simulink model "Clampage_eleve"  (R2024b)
settings: Solver=VariableStepAuto  StartTime=0.0  StopTime=1.5  MaxStep=1e-2  RelTol=1e-3  EnableMultiTasking=on
libraries: fl_lib x12, nesl_utility x5, simulink x2, ee_lib x2, simulink_extras x1

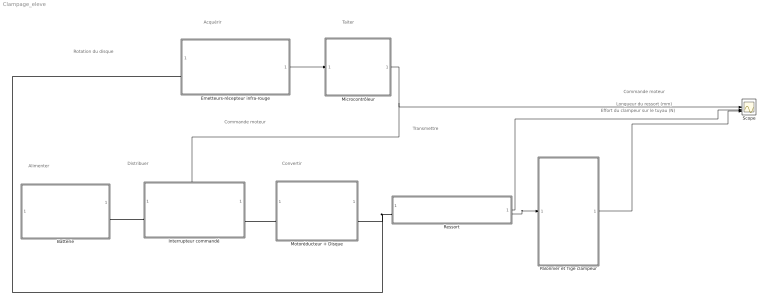
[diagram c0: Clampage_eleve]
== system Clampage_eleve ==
  note: Acquérir
  note: Longueur du ressort (mm)
  note: Effort du clampeur sur le tuyau (N)
  note: Commande moteur
  note: Taiter
  note: Convertir
  note: Alimenter
  note: Transmettre
  note: Rotation du disque
  note: Commande moteur
  note: Distribuer
  Batterie : Subsystem
  Emetteurs-récepteur infra-rouge : Subsystem
  Interrupteur commandé : Subsystem
  Microcontrôleur : Subsystem
  Motoréducteur + Disque : Subsystem  mask{V=0, R=0}
      mask prompts: V "Vitesse de rotation à vide (tr/min)"; R "Rapport de réduction"
  Palonnier et Tige clampeur : Subsystem
  Ressort : Subsystem  mask{k=0, L0=0}
      mask prompts: k "k : Raideur du ressort (N/mm)"; L0 "L0 : Longueur libre initiale du ressort (mm)"
  Scope : Scope  NumInputPorts=3
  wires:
  Ressort/2(Out3) -> Palonnier et Tige clampeur/1(In1)
  Emetteurs-récepteur infra-rouge/1(Out1) -> Microcontrôleur/1(S)
  Microcontrôleur/1(Q) -> Interrupteur commandé/1(In1), Scope/1
  Palonnier et Tige clampeur/1(Out1) -> Scope/3
  Ressort/1(Out1) -> Scope/2
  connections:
  Ressort/LConn1 -- Emetteurs-récepteur infra-rouge/LConn1 -- Motoréducteur + Disque/RConn1
  Interrupteur commandé/RConn1 -- Motoréducteur + Disque/LConn1
  Batterie/RConn1 -- Interrupteur commandé/LConn1

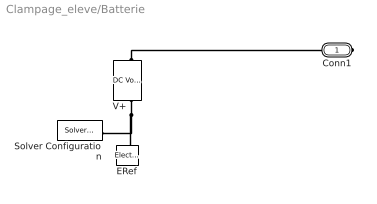
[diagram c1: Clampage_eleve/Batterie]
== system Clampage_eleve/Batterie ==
  ERef : fl_lib/Electrical/Electrical Elements/Electrical Reference
  Solver Configuration : nesl_utility/Solver Configuration  PhysicalDomain=network_engine_domain  SubClassName=solver  LeftPortType=input  RightPortType=generic  Tones=[]  Harmonics=[]  SimulateNoise=off  Profile=off  UseLocalSampling=off  EnableSwitchedLinearOptims=on  FrequencyDomain=off  UseCCode=off  RelTol=0.001  AbsTol=1e-06  MinStep=1e-09  ToWorkspace=off  RevertToSquareIcSolve=off  NumHomotopyIterations=100  PhasorMode=off  PhasorModeNumHarmonics=1  ConsistencySolver=NEWTON_FTOL  IndexReductionMethod=DerivativeReplacement  DoDC=off  ResidualTolerance=1e-9  ConsistencyTolSource=GLOBAL  ConsistencyAbsTol=0.001  ConsistencyRelTol=0.001  ConsistencyTolFactor=0.001  UseLocalSolver=off  LocalSolverChoice=NE_BACKWARD_EULER_ADVANCER  ResolveIndetEquations=on  FunctionEvalNumThread=1  LocalSolverSampleTime=.001  DoFixedCost=off  MaxNonlinIter=3  MaxModeIter=2  ComputeImpulses=off  ImpulseIterations=2  LinearAlgebra=auto  LinearAlgebraNumThread=0  EquationFormulation=NE_TIME_EF  DelaysMemoryBudget=1024  AutomaticFiltering=on  FilteringTimeConstant=0.001  PartitionStorageMethod=AS_NEEDED  PartitionMemoryBudget=1024  PartitionMethod=FAST  MultibodyUseLocalSolver=off  MultibodyLocalSolverChoice=ODE1  MultibodyLocalSolverSampleTime=0.001
  V+ : fl_lib/Electrical/Electrical Sources/DC Voltage Source  v0=12 V
  Conn1 : PMIOPort  Side=Right
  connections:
  V+/RConn1 -- ERef/LConn1 -- Solver Configuration/RConn1
  V+/LConn1 -- Conn1/RConn1

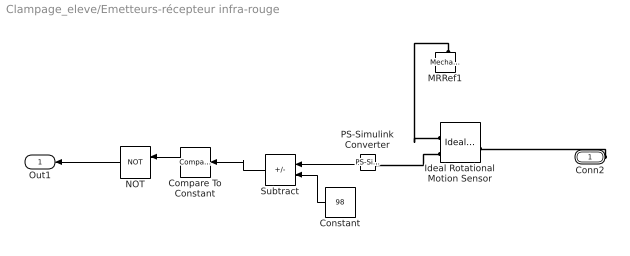
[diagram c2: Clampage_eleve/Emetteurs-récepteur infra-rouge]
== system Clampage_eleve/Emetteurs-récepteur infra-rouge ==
  Compare To Constant : simulink/Logic and Bit Operations/Compare To Constant  relop=<=  const=0  OutDataTypeStr=uint8
  Constant : Constant  Value=98
  Ideal Rotational Motion Sensor : fl_lib/Mechanical/Mechanical Sensors/Ideal Rotational Motion Sensor  reference=foundation.enum.MeasurementReference.difference  acceleration_port=false  velocity_port=true  position_port=true  wrap_angle=false  offset=0 rad
  MRRef1 : fl_lib/Mechanical/Rotational Elements/Mechanical Rotational Reference
  NOT : Logic  Operator=NOT  IconShape=distinctive  AllPortsSameDT=off  OutDataTypeStr=boolean
  PS-Simulink Converter : nesl_utility/PS-Simulink Converter  PhysicalDomain=network_engine_domain  SubClassName=ps_output  LeftPortType=input  RightPortType=output  PseudoPeriodic=off  Frequencies=[]  VectorFormat=inherit  Unit=deg  AffineConversion=off
  Subtract : Sum  Inputs=+-
  Conn2 : PMIOPort  Side=Left
  Out1 : Outport
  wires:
  Constant/1 -> Subtract/2
  Subtract/1 -> Compare To Constant/1
  Compare To Constant/1 -> NOT/1
  PS-Simulink Converter/1 -> Subtract/1
  NOT/1 -> Out1/1
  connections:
  Ideal Rotational Motion Sensor/RConn3 -- PS-Simulink Converter/LConn1
  MRRef1/LConn1 -- Ideal Rotational Motion Sensor/RConn1
  Ideal Rotational Motion Sensor/LConn1 -- Conn2/RConn1

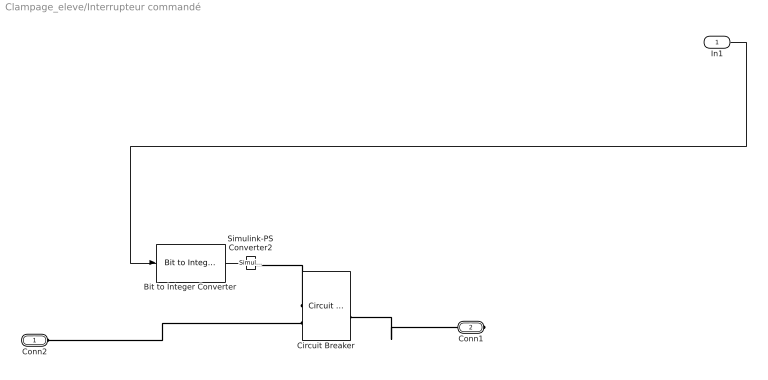
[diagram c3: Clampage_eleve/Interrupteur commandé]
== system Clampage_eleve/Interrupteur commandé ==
  In1 : Inport
  Bit to Integer Converter : simulink/Logic and Bit Operations/Bit to Integer Converter  nbits=1  bitOrder=MSB first  signedOutputValues=Unsigned  outDtype=double  outDtypeSigned=Inherit via internal rule
  Circuit Breaker : ee_lib/Switches & Breakers/Circuit Breaker  R_closed=0.001 Ohm  G_open=1e-6 1/Ohm  threshold=0.5 V  breaker_behavior=ee.enum.switches.breakerBehavior.zeroCrossingDisable
  Simulink-PS Converter2 : nesl_utility/Simulink-PS Converter  PhysicalDomain=network_engine_domain  SubClassName=ps_input  LeftPortType=input  RightPortType=output  PseudoPeriodic=off  Frequencies=[]  NoiseDistribution=none  NoiseParameters=[]  Unit=1  AffineConversion=off  FilteringAndDerivatives=provide  SimscapeFilterOrder=1  InputFilterTimeConstant=0.001  UdotUserProvided=0
  Conn2 : PMIOPort  Side=Left
  Conn1 : PMIOPort  Port=2  Side=Right
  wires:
  Bit to Integer Converter/1 -> Simulink-PS Converter2/1
  In1/1 -> Bit to Integer Converter/1
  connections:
  Circuit Breaker/LConn1 -- Simulink-PS Converter2/RConn1
  Circuit Breaker/RConn1 -- Conn1/RConn1
  Conn2/RConn1 -- Circuit Breaker/LConn2

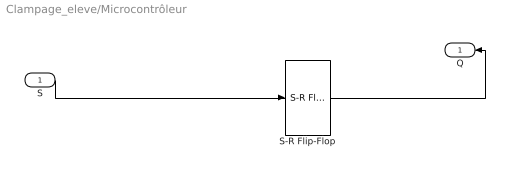
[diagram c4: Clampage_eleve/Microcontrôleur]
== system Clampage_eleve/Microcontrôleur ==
  S : Inport
  S-R Flip-Flop : simulink_extras/Flip Flops/S-R Flip-Flop  initial_condition=0
  Q : Outport
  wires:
  S-R Flip-Flop/1 -> Q/1
  S/1 -> S-R Flip-Flop/1

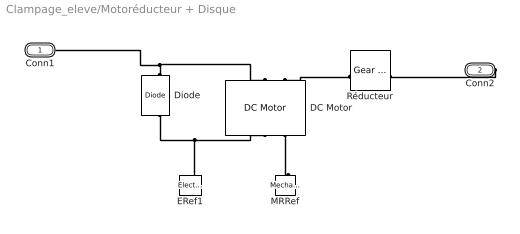
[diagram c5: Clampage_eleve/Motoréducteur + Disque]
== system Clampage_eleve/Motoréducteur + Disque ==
  DC Motor : ee_lib/Electromechanical/Brushed Motors/DC Motor  field_option=ee.enum.field_option.pm  Rf=100 Ohm  Lf=1 H  Laf=0.15 H  If0=0 A  parameterization=ee.enum.dcparam_option.load_speed  Ra=20.6 Ohm  La=1.13 mH  emf_or_torque=ee.enum.emf_or_torque.kv  Kv=0.00146 V/rpm  Ki=14 m*mN/A  T_stall=3e-3*4000/(2*pi*6.25) N*m  w_max=V rpm  w_rated=2570 rpm  P_rated=2.5 W  V_rated=9 V  lam_param=ee.enum.lam_param.current  i_noload=12 mA  V_i_noload=9 V  J=0.3 cm^2*g  lam=1e-08 N*m/(rad/s)  speed0=5870 rpm  t_fault_armature=1 s  t_fault_field=1 s  fault_action=simscape.enum.assert.action.none  alpha=3.93e-3 1/K  Tmeas=25 degC  thermal_mass=100 J/K  initial_temperature=25 degC
  Diode : fl_lib/Electrical/Electrical Elements/Diode  Vf=0.6 V  Ron=0.3 Ohm  Goff=1e-8 1/Ohm  i_specify=off  i_priority=None  i=0 A  i_nominal_specify=off  i_nominal_value=1  i_nominal_unit=A  v_specify=off  v_priority=None  v=0 V  v_nominal_specify=off  v_nominal_value=1  v_nominal_unit=V
  ERef1 : fl_lib/Electrical/Electrical Elements/Electrical Reference
  MRRef : fl_lib/Mechanical/Rotational Elements/Mechanical Rotational Reference
  Réducteur : fl_lib/Mechanical/Mechanisms/Gear Box  ratio=R  t_in_specify=off  t_in_priority=None  t_in=0 N*m  t_in_nominal_specify=off  t_in_nominal_value=1  t_in_nominal_unit=N*m  t_out_specify=off  t_out_priority=None  t_out=0 N*m  t_out_nominal_specify=off  t_out_nominal_value=1  t_out_nominal_unit=N*m
  Conn1 : PMIOPort  Side=Left
  Conn2 : PMIOPort  Port=2  Side=Right
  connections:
  DC Motor/RConn2 -- MRRef/LConn1
  Réducteur/LConn1 -- DC Motor/LConn2
  Conn2/RConn1 -- Réducteur/RConn1
  Diode/LConn1 -- ERef1/LConn1 -- DC Motor/RConn1
  Diode/RConn1 -- Conn1/RConn1 -- DC Motor/LConn1

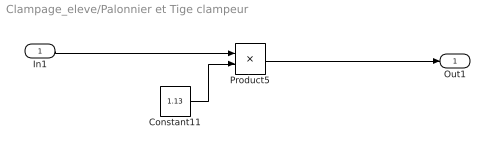
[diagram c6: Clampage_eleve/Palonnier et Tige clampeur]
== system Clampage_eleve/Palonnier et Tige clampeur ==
  In1 : Inport
  Constant11 : Constant  Value=1.13
  Product5 : Product
  Out1 : Outport
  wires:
  Constant11/1 -> Product5/2
  Product5/1 -> Out1/1
  In1/1 -> Product5/1

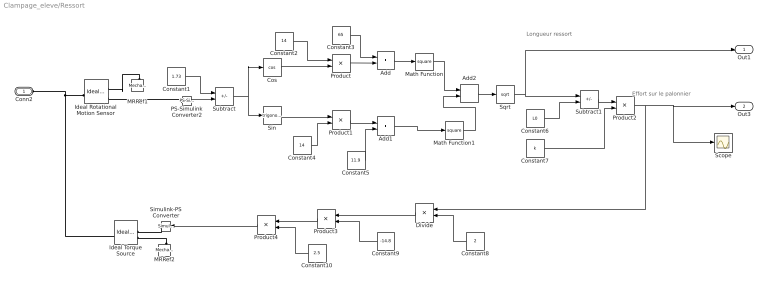
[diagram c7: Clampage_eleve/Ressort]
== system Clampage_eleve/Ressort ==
  note: Effort sur le palonnier
  note: Longueur ressort
  Add : Sum
  Add1 : Sum
  Add2 : Sum
  Constant1 : Constant  Value=1.73
  Constant10 : Constant  Value=2.5
  Constant2 : Constant  Value=14
  Constant3 : Constant  Value=65
  Constant4 : Constant  Value=14
  Constant5 : Constant  Value=11.9
  Constant6 : Constant  Value=L0
  Constant7 : Constant  Value=k
  Constant8 : Constant  Value=2
  Constant9 : Constant  Value=-14.8
  Cos : Trigonometry  Operator=cos  OutputSignalType=real
  Divide : Product  Inputs=*/
  Ideal Rotational Motion Sensor : fl_lib/Mechanical/Mechanical Sensors/Ideal Rotational Motion Sensor  reference=foundation.enum.MeasurementReference.difference  acceleration_port=false  velocity_port=true  position_port=true  wrap_angle=false  offset=0 rad
  Ideal Torque Source : fl_lib/Mechanical/Mechanical Sources/Ideal Torque Source
  MRRef1 : fl_lib/Mechanical/Rotational Elements/Mechanical Rotational Reference
  MRRef2 : fl_lib/Mechanical/Rotational Elements/Mechanical Rotational Reference
  Math Function : Math  Operator=square
  Math Function1 : Math  Operator=square
  PS-Simulink Converter2 : nesl_utility/PS-Simulink Converter  PhysicalDomain=network_engine_domain  SubClassName=ps_output  LeftPortType=input  RightPortType=output  PseudoPeriodic=off  Frequencies=[]  VectorFormat=1-D array  Unit=rad  AffineConversion=off
  Product{,1..4} (5 alike) : Product
  Scope : Scope
  Simulink-PS Converter : nesl_utility/Simulink-PS Converter  PhysicalDomain=network_engine_domain  SubClassName=ps_input  LeftPortType=input  RightPortType=output  PseudoPeriodic=off  Frequencies=[]  NoiseDistribution=none  NoiseParameters=[]  Unit=mN*m  AffineConversion=off  FilteringAndDerivatives=provide  SimscapeFilterOrder=1  InputFilterTimeConstant=0.001  UdotUserProvided=0
  Sin : Trigonometry  OutputSignalType=real
  Sqrt : Sqrt
  Subtract : Sum  Inputs=+-
  Subtract1 : Sum  Inputs=+-
  Conn2 : PMIOPort  Side=Left
  Out1 : Outport
  Out3 : Outport  Port=2
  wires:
  Add/1 -> Math Function/1
  Add2/1 -> Sqrt/1
  Divide/1 -> Product3/1
  Product4/1 -> Simulink-PS Converter/1
  Subtract/1 -> Cos/1, Sin/1
  Constant8/1 -> Divide/2
  Cos/1 -> Product/2
  Math Function1/1 -> Add2/2
  Constant2/1 -> Product/1
  Constant1/1 -> Subtract/1
  Product2/1 -> Divide/1, Scope/1, Out3/1
  Constant5/1 -> Add1/2
  Constant4/1 -> Product1/2
  Add1/1 -> Math Function1/1
  Math Function/1 -> Add2/1
  Sqrt/1 -> Out1/1, Subtract1/1
  Product3/1 -> Product4/1
  Product1/1 -> Add1/1
  PS-Simulink Converter2/1 -> Subtract/2
  Constant3/1 -> Add/1
  Sin/1 -> Product1/1
  Product/1 -> Add/2
  Subtract1/1 -> Product2/1
  Constant9/1 -> Product3/2
  Constant10/1 -> Product4/2
  Constant6/1 -> Subtract1/2
  Constant7/1 -> Product2/2
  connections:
  Simulink-PS Converter/RConn1 -- Ideal Torque Source/RConn1
  MRRef1/LConn1 -- Ideal Rotational Motion Sensor/RConn1
  Ideal Rotational Motion Sensor/LConn1 -- Conn2/RConn1 -- Ideal Torque Source/LConn1
  PS-Simulink Converter2/LConn1 -- Ideal Rotational Motion Sensor/RConn3
  MRRef2/LConn1 -- Ideal Torque Source/RConn2
